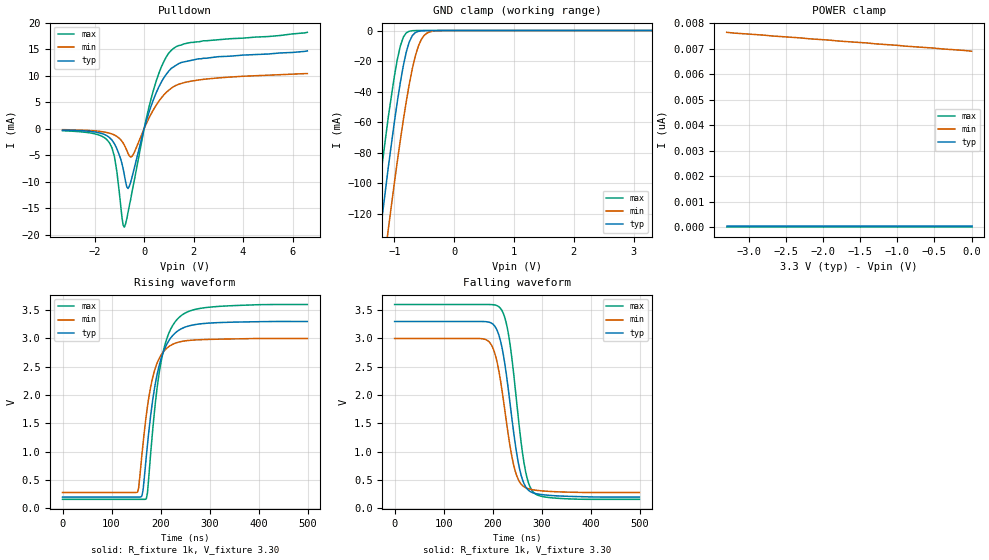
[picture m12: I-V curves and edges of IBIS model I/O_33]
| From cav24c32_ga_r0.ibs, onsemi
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|//////////////////////////////////////////////////////////////////////////////
|//////////////////////////////////////////////////////////////////////////////
[Model] I/O_33
Model_type I/O_open_drain
Vinh = 2.31
Vinl = 0.99
Vmeas = 1.65
Vref = 3.30
Rref = 1000
Cref = 0pF
|  variable   typ   min   max
C_comp   8pF   8pF   8pF
|//////////////////////////////////////////////////////////////////////////////
[Temperature Range]   25   125   -40
|//////////////////////////////////////////////////////////////////////////////
[Voltage Range]   3.30V   3.00V   3.60V
|//////////////////////////////////////////////////////////////////////////////
[Pulldown Reference]   0V   0V   0V
|//////////////////////////////////////////////////////////////////////////////
[POWER Clamp Reference] 3.30V   3.00V   3.60V
|//////////////////////////////////////////////////////////////////////////////
[GND Clamp Reference]   0V   0V   0V
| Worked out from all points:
|   slope of the pulldown table from 0 to 0.495 V, typ, clamps not added: 72.2 ohm
|   GND clamp passes 1 mA (typ) near -0.63 V on its own axis
|   falling waveform, R_fixture 1k, V_fixture 3.30: 20-80 % time 29.6ns typ, 29.4ns min, 28ns max; typ from 3.3 V to 0.2 V
|   rising waveform, R_fixture 1k, V_fixture 3.30: 20-80 % time 32.5ns typ, 27.9ns min, 31ns max; typ from 0.2 V to 3.3 V
|//////////////////////////////////////////////////////////////////////////////
[Pulldown]
|   Voltage   I(typ)   I(min)   I(max)
-3.3V     -246uA     -182uA     -392uA
-1.4V     -1.67mA    -850uA     -2.68mA
-1.2V     -2.85mA    -1.2mA     -5.29mA
-900mV    -6.52mA    -2.35mA    -16.6mA
-800mV    -8.74mA    -3.09mA    -18.6mA
-700mV    -11mA      -4.11mA    -17mA
-600mV    -10.9mA    -5.13mA    -14.6mA
-450mV    -8.43mA    -4.96mA    -11mA
300mV     4.51mA     2.94mA     5.98mA
700mV     8.83mA     5.83mA     11.7mA
1.1V      11.4mA     7.65mA     14.8mA
6.6V      14.7mA     10.4mA     18.2mA
|//////////////////////////////////////////////////////////////////////////////
[GND Clamp]
|   Voltage   I(typ)   I(min)   I(max)
-3.3V     -2.04A     -1.82A     -2.22A
-1.3V     -162mA     -199mA     -135mA
-1.2V     -121mA     -162mA     -86.7mA
-1.1V     -89.4mA    -130mA     -56.4mA
-1V       -60.1mA    -100mA     -30.1mA
-900mV    -34.1mA    -71.9mA    -10.2mA
-850mV    -23.1mA    -58.7mA    -4.35mA
-750mV    -7.4mA     -35.1mA    -451uA
-600mV    -540uA     -10.4mA    -10.1uA
-500mV    -75.3uA    -3.13mA    -790nA
-400mV    -10.3uA    -773uA     -61.5nA
3.3V      30pA       6.97nA     266fA
|//////////////////////////////////////////////////////////////////////////////
[POWER Clamp]
|   Voltage   I(typ)   I(min)   I(max)
-3.3V     30pA       7.64nA     266fA
-3.2V     30pA       7.61nA     266fA
-2.8V     30pA       7.53nA     266fA
-2.7V     30pA       7.5nA      266fA
-1.9V     30pA       7.33nA     266fA
-1.8V     30pA       7.3nA      266fA
-1.4V     30pA       7.22nA     266fA
-1.3V     30pA       7.19nA     266fA
-1V       30pA       7.13nA     266fA
-900mV    30pA       7.1nA      266fA
-500mV    30pA       7.02nA     266fA
0V        30pA       6.9nA      266fA
|//////////////////////////////////////////////////////////////////////////////
|//////////////////////////////////////////////////////////////////////////////
[Ramp]
|  variable   typ   min   max
dV/dt_r   1.860E+00/3.150E-08  1.632E+00/2.700E-08  2.064E+00/3.150E-08
dV/dt_f   1.860E+00/3.000E-08  1.632E+00/3.000E-08  2.064E+00/2.700E-08
R_load = 1k
|/////////////////////////////////////////////////////////////////////////////
[Falling Waveform]
R_fixture = 1k
V_fixture = 3.30
V_fixture_min = 3.00
V_fixture_max = 3.60
C_fixture = 0p
|   time   V(typ)   V(min)   V(max)
0s        3.3V       3V         3.6V
186ns     3.297V     2.981V     3.6V
201ns     3.25V      2.823V     3.596V
213ns     3.053V     2.413V     3.559V
231ns     2.17V      1.354V     3.141V
246ns     1.147V     661.7mV    2.129V
255ns     695.6mV    466.9mV    1.394V
264ns     437.2mV    381.7mV    804.7mV
282ns     275.8mV    328.8mV    296.5mV
499.5ns   200mV      280mV      160mV
|//////////////////////////////////////////////////////////////////////////////
[Rising Waveform]
R_fixture = 1k
V_fixture = 3.30
V_fixture_min = 3.00
V_fixture_max = 3.60
C_fixture = 0p
|   time   V(typ)   V(min)   V(max)
0s        200mV      280mV      160mV
153ns     200mV      286.3mV    160mV
162ns     219mV      948.2mV    160mV
171ns     923.4mV    1.652V     171.3mV
184.5ns   1.944V     2.33V      1.436V
193.5ns   2.387V     2.576V     2.163V
202.5ns   2.682V     2.726V     2.652V
220.5ns   3.007V     2.877V     3.162V
243ns     3.174V     2.948V     3.409V
499.5ns   3.3V       3V         3.6V
